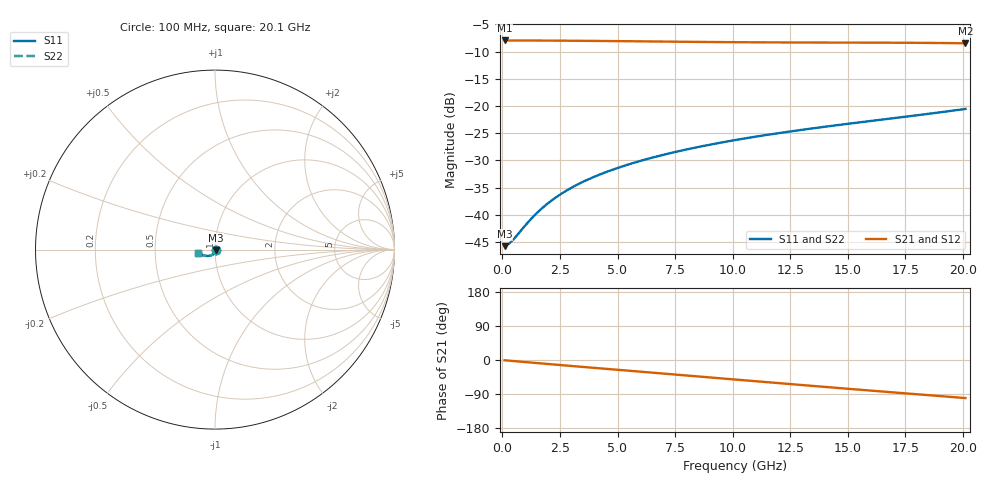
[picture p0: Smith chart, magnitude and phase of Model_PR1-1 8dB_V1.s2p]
!version-1
!date-07.2020
!Series
#	GHZ S RI R 50.0
!	FREQ.GHZ	S11RE	S11IM	S21RE	S21IM	S12RE	S12IM	S22RE	S22IM
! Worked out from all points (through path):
!   101 points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, 100 MHz to 20.1 GHz, reference 50 ohm
!   highest |S21| = -7.96 dB at 100 MHz (marker M1); lowest = -8.5 dB at 20.1 GHz (marker M2)
!   group delay of S21, straight-line fit = 13.9 ps
!   lowest |S11| = -45.7 dB at 100 MHz (marker M3), VSWR 1.01, Z = 50.5 - j0.138 ohm
!   |S11| at or under -10 dB: start of sweep to end of sweep
!   |S22| runs from -45.7 to -20.5 dB; largest |S21 - S12| = 0
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0.1  0.00498 -0.00137  0.3999 -0.00475  0.3999 -0.00475  0.00498 -0.00137
0.3  0.00473 -0.00272  0.3997 -0.0122  0.3997 -0.0122  0.00473 -0.00272
0.5  0.00444 -0.00405  0.3994 -0.0196  0.3994 -0.0196  0.00444 -0.00405
1.1  0.00337 -0.00779  0.3973 -0.0416  0.3973 -0.0416  0.00337 -0.00779
1.3  0.00295 -0.00896  0.3964 -0.0488  0.3964 -0.0488  0.00295 -0.00896
1.5  0.00249 -0.0101  0.3953 -0.0559  0.3953 -0.0559  0.00249 -0.0101
1.9  0.00149 -0.0123  0.3927 -0.0701  0.3927 -0.0701  0.00149 -0.0123
2.3  0.000377 -0.0143  0.3895 -0.084  0.3895 -0.084  0.000377 -0.0143
2.7  -0.00084 -0.0163  0.3858 -0.0977  0.3858 -0.0977  -0.00084 -0.0163
3.5  -0.00355 -0.0198  0.3769 -0.1245  0.3769 -0.1245  -0.00355 -0.0198
4.3  -0.00659 -0.0229  0.366 -0.1502  0.366 -0.1502  -0.00659 -0.0229
5.1  -0.00989 -0.0256  0.3533 -0.1748  0.3533 -0.1748  -0.00989 -0.0256
5.9  -0.0134 -0.0279  0.3389 -0.1984  0.3389 -0.1984  -0.0134 -0.0279
6.9  -0.0181 -0.0303  0.3187 -0.2262  0.3187 -0.2262  -0.0181 -0.0303
8.5  -0.0259 -0.0331  0.2818 -0.2666  0.2818 -0.2666  -0.0259 -0.0331
10.1  -0.034 -0.0348  0.2401 -0.3017  0.2401 -0.3017  -0.034 -0.0348
11.9  -0.0434 -0.0353  0.1888 -0.3341  0.1888 -0.3341  -0.0434 -0.0353
13.5  -0.0519 -0.0347  0.1402 -0.3562  0.1402 -0.3562  -0.0519 -0.0347
15.3  -0.0618 -0.0327  0.0835 -0.3729  0.0835 -0.3729  -0.0618 -0.0327
16.9  -0.0711 -0.0295  0.0323 -0.3799  0.0323 -0.3799  -0.0711 -0.0295
18.5  -0.0811 -0.025  -0.0186 -0.3793  -0.0186 -0.3793  -0.0811 -0.025
20.1  -0.0922 -0.0187  -0.0683 -0.3704  -0.0683 -0.3704  -0.0922 -0.0187
